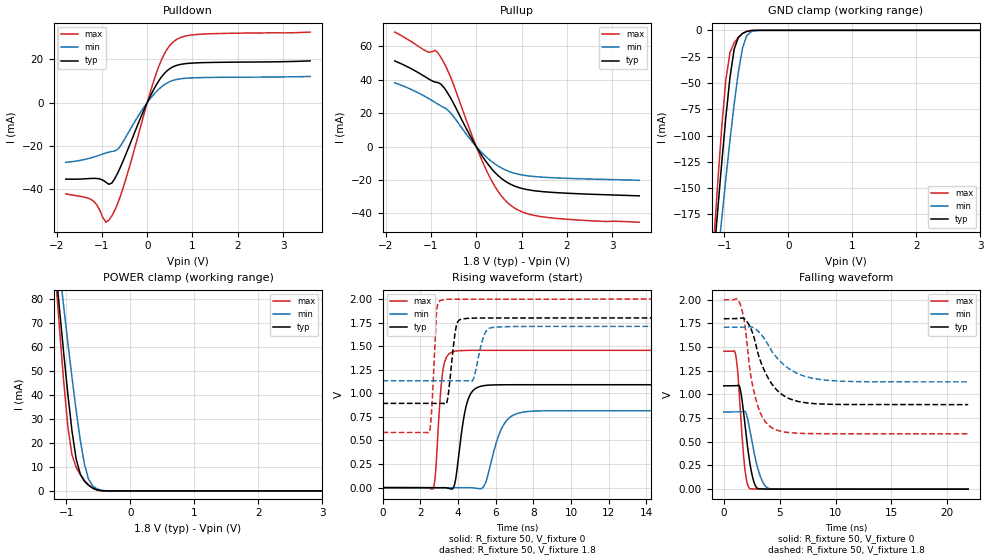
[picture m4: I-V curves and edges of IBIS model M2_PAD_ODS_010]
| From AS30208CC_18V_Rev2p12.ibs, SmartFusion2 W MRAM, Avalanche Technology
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[Model] M2_PAD_ODS_010
Model_type I/O
Enable   Active-High
Vinl  =  0.63
Vinh  =  1.17
Vmeas =  0.9
Cref  =  30e-12
| Capacitance  typ   min   max
C_comp   1.627116e-12   1.521588e-12   1.744735e-12
| Variables   typ   min   max
[GND Clamp Reference]   0   0   0
[POWER Clamp Reference]   1.8   1.71   2
[Pulldown Reference]   0   0   0
[Pullup Reference]   1.8   1.71   2
[Temperature Range]   25   125   -40
[Voltage Range]   1.8   1.71   2
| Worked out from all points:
|   slope of the pulldown table from 0 to 0.27 V, typ, clamps not added: 25.7 ohm
|   slope of the pullup table from 0 to 0.27 V, typ, clamps not added: 24.7 ohm
|   GND clamp passes 1 mA (typ) near -0.64 V on its own axis
|   POWER clamp passes 1 mA (typ) near -0.57 V on its own axis
|   falling waveform, R_fixture 50, V_fixture 0: 20-80 % time 705ps typ, 900ps min, 525ps max; typ from 1.09 V to 0 V
|   falling waveform, R_fixture 50, V_fixture 1.8: 20-80 % time 1.87ns typ, 2.55ns min, 1.16ns max; typ from 1.8 V to 0.893 V
|   rising waveform, R_fixture 50, V_fixture 0: 20-80 % time 478ps typ, 757ps min, 293ps max; typ from 0 V to 1.09 V
|   rising waveform, R_fixture 50, V_fixture 1.8: 20-80 % time 293ps typ, 401ps min, 204ps max; typ from 0.893 V to 1.8 V
[GND Clamp]
| Voltage   I(typ)   I(min)   I(max)
-1.8V     -720.5mA   -670.5mA   -825.4mA
-1.173V   -222.3mA   -260.3mA   -207.7mA
-1.108V   -173.8mA   -219.8mA   -148.5mA
-1.043V   -127mA     -180.1mA   -93.3mA
-977.6mV  -83.06mA   -141.5mA   -47.19mA
-912.4mV  -44.72mA   -104.6mA   -21.23mA
-847.2mV  -17.99mA   -70.1mA    -11.92mA
-782.1mV  -6.766mA   -39.85mA   -6.657mA
-716.9mV  -2.938mA   -17.13mA   -3.048mA
-651.7mV  -1.119mA   -5.25mA    -952uA
-456.2mV  -3.98uA    -74.41uA   -422.2nA
3.6V      0A         0A         0A
[POWER Clamp]
| Voltage   I(typ)   I(min)   I(max)
-1.8V     287.1mA    268.3mA    329.6mA
-1.173V   94.89mA    108.5mA    91.02mA
-1.108V   76.1mA     92.66mA    67.97mA
-1.043V   57.9mA     77.16mA    46.14mA
-977.6mV  40.62mA    62.05mA    27.14mA
-912.4mV  25.13mA    47.46mA    15.06mA
-847.2mV  13.38mA    33.64mA    9.853mA
-716.9mV  4.014mA    11.09mA    4.394mA
-651.7mV  2.34mA     4.821mA    2.483mA
-586.6mV  1.18mA     2.003mA    1.113mA
-325.9mV  1.153uA    19.85uA    110.1nA
3.6V      0A         0A         0A
[Pulldown]
| Voltage   I(typ)   I(min)   I(max)
-1.8V     -35.45mA   -27.68mA   -42.34mA
-1.238V   -35.17mA   -25.59mA   -44.93mA
-912.4mV  -36.92mA   -23.37mA   -55.44mA
-847.2mV  -37.89mA   -22.97mA   -54.5mA
-716.9mV  -35.26mA   -22.46mA   -49.94mA
-521.4mV  -26.49mA   -17.75mA   -38.78mA
-65.17mV  -3.048mA   -1.907mA   -4.891mA
248.3mV   9.844mA    6.047mA    16.33mA
434.5mV   14.66mA    9.037mA    24.58mA
620.7mV   17.01mA    10.57mA    28.86mA
1.179V    18.47mA    11.56mA    31.67mA
3.6V      19.32mA    12.09mA    32.66mA
[Pullup]
| Voltage   I(typ)   I(min)   I(max)
-1.8V     51.26mA    38.2mA     68.51mA
-1.108V   41.41mA    29.63mA    57.12mA
-912.4mV  38.62mA    26.49mA    57.6mA
-782.1mV  37.38mA    24.37mA    53.47mA
-586.6mV  30.05mA    20.74mA    42.91mA
-65.17mV  3.056mA    2.089mA    4.574mA
248.3mV   -10.17mA   -6.821mA   -15.55mA
496.6mV   -17.67mA   -11.85mA   -27.35mA
744.8mV   -22.35mA   -15.08mA   -34.79mA
1.055V    -25.34mA   -17.17mA   -39.5mA
1.49V     -26.99mA   -18.33mA   -42.12mA
3.6V      -29.46mA   -20.13mA   -45.23mA
[Ramp]
dV/dt_r   0.654716/0.478038n  0.48928/0.757289n  0.873693/0.293466n
dV/dt_f   0.544072/1.87428n  0.34603/2.55073n  0.848875/1.16213n
R_load = 50
[Falling Waveform]
R_fixture = 50
V_fixture = 0
V_fixture_min = 0
V_fixture_max = 0
| Time   V(typ)   V(min)   V(max)
0s        1.091V     815.5mV    1.456V
1.06ns    1.092V     815.8mV    1.419V
1.213ns   1.094V     815.8mV    1.284V
1.441ns   1.072V     815.9mV    904.9mV
1.842ns   738.2mV    823.1mV    265.2mV
2.062ns   508.9mV    777.9mV    77.1mV
2.304ns   296.7mV    643.9mV    6.371mV
2.909ns   19.87mV    280.8mV    1.126mV
3.944ns   1.148mV    11.31mV    538.8uV
21.88ns   518.6nV    1.466uV    84.12nV
[Falling Waveform]
R_fixture = 50
V_fixture = 1.8
V_fixture_min = 1.71
V_fixture_max = 2
| Time   V(typ)   V(min)   V(max)
0s        1.8V       1.71V      2V
1.428ns   1.806V     1.711V     1.965V
1.827ns   1.8V       1.711V     1.784V
2.349ns   1.715V     1.716V     1.25V
2.816ns   1.553V     1.694V     972.4mV
3.476ns   1.293V     1.615V     755.2mV
4.333ns   1.106V     1.452V     645.7mV
5.928ns   952.8mV    1.265V     596.3mV
8.089ns   903.4mV    1.168V     586.3mV
21.88ns   893.2mV    1.133V     585.2mV
[Rising Waveform]
R_fixture = 50
V_fixture = 0
V_fixture_min = 0
V_fixture_max = 0
| Time   V(typ)   V(min)   V(max)
0s        2.043nV    50.02nV    113nV
2.684ns   -290.6uV   -489uV     -11.54mV
2.809ns   -304.1uV   -511.8uV   149.5mV
3.201ns   -346.6uV   -583.3uV   1.243V
3.747ns   -4.679mV   -682.6uV   1.443V
4.448ns   875.7mV    -810.5uV   1.455V
5.236ns   1.077V     -10.41mV   1.456V
6.304ns   1.091V     621.9mV    1.456V
7.412ns   1.091V     799.5mV    1.456V
21.88ns   1.091V     815.5mV    1.456V
[Rising Waveform]
R_fixture = 50
V_fixture = 1.8
V_fixture_min = 1.71
V_fixture_max = 2
| Time   V(typ)   V(min)   V(max)
0s        893.2mV    1.133V     585.2mV
2.48ns    894mV      1.134V     589.5mV
2.873ns   894.1mV    1.134V     1.869V
3.131ns   894.2mV    1.134V     1.989V
3.428ns   916.6mV    1.134V     1.997V
3.862ns   1.66V      1.134V     1.999V
4.233ns   1.789V     1.134V     1.999V
4.78ns    1.798V     1.136V     1.999V
5.793ns   1.799V     1.697V     1.999V
21.88ns   1.8V       1.71V      2V
